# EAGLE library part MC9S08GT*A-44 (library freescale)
HCS08 Microcontroller Source: http://www.freescale.com/files/microcontrollers/doc/data_sheet/MC9S08GT16A.pdf
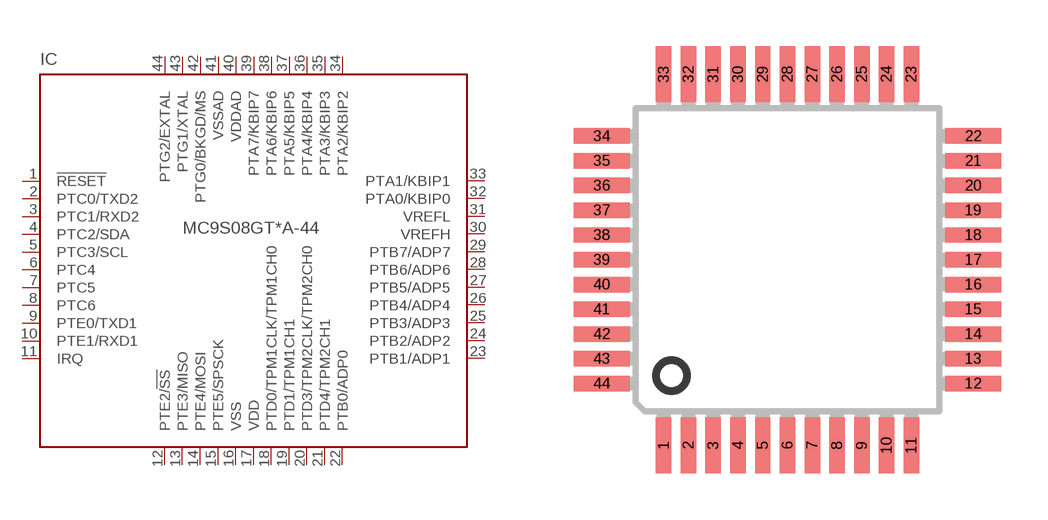
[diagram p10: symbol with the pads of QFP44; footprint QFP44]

Designator prefix IC

## MC9S08GT16A-44 (MF: MOTOROLA; MPN: MC9S08GT16ACFBE; OC_FARNELL: 1579706; OC_NEWARK: 01M5859), MC9S08GT8A-44 (MF: MOTOROLA; MPN: MC9S08GT8AMFBE; OC_FARNELL: 1294361; OC_NEWARK: 01M5872)  [QFP44]
1  !RESET  in
2  PTC0/TXD2
3  PTC1/RXD2
4  PTC2/SDA
5  PTC3/SCL
6  PTC4
7  PTC5
8  PTC6
9  PTE0/TXD1
10  PTE1/RXD1
11  IRQ
12  PTE2/!SS
13  PTE3/MISO
14  PTE4/MOSI
15  PTE5/SPSCK
16  VSS  pwr
17  VDD  pwr
18  PTD0/TPM1CLK/TPM1CH0
19  PTD1/TPM1CH1
20  PTD3/TPM2CLK/TPM2CH0
21  PTD4/TPM2CH1
22  PTB0/ADP0
23  PTB1/ADP1
24  PTB2/ADP2
25  PTB3/ADP3
26  PTB4/ADP4
27  PTB5/ADP5
28  PTB6/ADP6
29  PTB7/ADP7
30  VREFH
31  VREFL
32  PTA0/KBIP0
33  PTA1/KBIP1
34  PTA2/KBIP2
35  PTA3/KBIP3
36  PTA4/KBIP4
37  PTA5/KBIP5
38  PTA6/KBIP6
39  PTA7/KBIP7
40  VDDAD  pwr
41  VSSAD  pwr
42  PTG0/BKGD/MS
43  PTG1/XTAL
44  PTG2/EXTAL

## Footprint QFP44 (pad centres in mm)
44-Pin QFP (Case #824A) Source: http://www.freescale.com/files/microcontrollers/doc/data_sheet/MC68HC908AP64.pdf
smd 0.5 x 1.8: 1 -4,-6; 2 -3.2,-6; 3 -2.4,-6; 4 -1.6,-6; 5 -0.8,-6; 6 0,-6; 7 0.8,-6; 8 1.6,-6; 9 2.4,-6; 10 3.2,-6; 11 4,-6; 23 4,6; 24 3.2,6; 25 2.4,6; 26 1.6,6; 27 0.8,6; 28 0,6; 29 -0.8,6; 30 -1.6,6; 31 -2.4,6; 32 -3.2,6; 33 -4,6
smd 1.8 x 0.5: 12 6,-4; 13 6,-3.2; 14 6,-2.4; 15 6,-1.6; 16 6,-0.8; 17 6,0; 18 6,0.8; 19 6,1.6; 20 6,2.4; 21 6,3.2; 22 6,4; 34 -6,4; 35 -6,3.2; 36 -6,2.4; 37 -6,1.6; 38 -6,0.8; 39 -6,0; 40 -6,-0.8; 41 -6,-1.6; 42 -6,-2.4; 43 -6,-3.2; 44 -6,-4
